PROGRAM MAIN
VAR
	stEl5131						:	ST_EL5131;
	fbEL5131_SingleCycle			:	FB_EL5131_SingleCycle;
	bSetCounter						:	BOOL;
	nSetCounterValue				:	UDINT := 0;
	bReset							:	BOOL;
	bRun							:	BOOL;
END_VAR

	
	fbEL5131_SingleCycle(
		bSetCounter:= bSetCounter, 
		nSetCounterValue:= nSetCounterValue, 
		bReset:= bReset, 
		bRun:= bRun,
		stEl5131:= stEl5131,
		bInited=> );

END_PROGRAM
